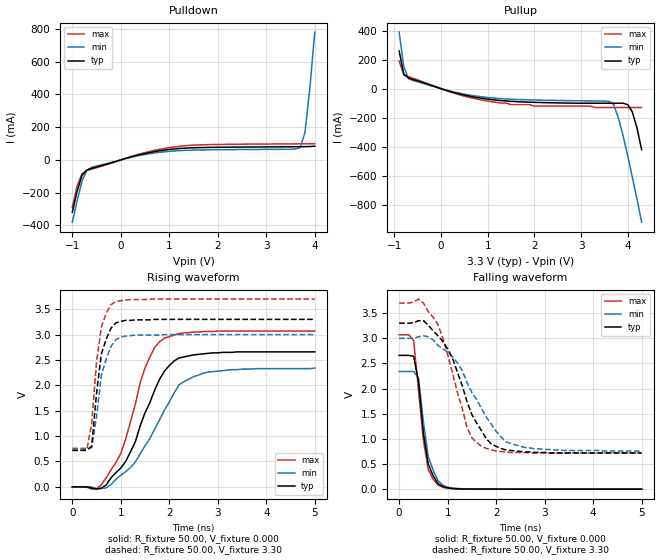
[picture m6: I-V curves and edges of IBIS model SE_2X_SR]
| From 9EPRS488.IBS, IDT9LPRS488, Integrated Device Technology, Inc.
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|   Model SE_2X_SR
[Model]   SE_2X_SR
Model_type   Output
Polarity   Inverting
Vmeas =   1.50V
Cref =   5.00pF
Rref =  0.000
Vref =   1.50V
C_comp   3.40pF   2.85pF   3.95pF
[Temperature Range]   27.00   70.00   0.000
[Voltage Range]   3.30V   3.00V   3.70V
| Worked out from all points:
|   slope of the pulldown table from 0 to 0.495 V, typ, clamps not added: 12.7 ohm
|   slope of the pullup table from 0 to 0.495 V, typ, clamps not added: 11.3 ohm
|   rising waveform, R_fixture 50.00, V_fixture 0.000: 20-80 % time 688ps typ, 834ps min, 578ps max; typ from 0 V to 2.66 V
|   rising waveform, R_fixture 50.00, V_fixture 3.30: 20-80 % time 215ps typ, 241ps min, 187ps max; typ from 0.72 V to 3.3 V
|   falling waveform, R_fixture 50.00, V_fixture 0.000: 20-80 % time 195ps typ, 229ps min, 211ps max; typ from 2.66 V to 0 V
|   falling waveform, R_fixture 50.00, V_fixture 3.30: 20-80 % time 646ps typ, 794ps min, 514ps max; typ from 3.3 V to 0.72 V
[Pulldown]
| voltage   I(typ)   I(min)   I(max)
|  -3.30   -4.16A   -4.01A   -4.26A
|  -3.10   -3.82A   -3.69A   -3.90A
|  -2.90   -3.48A   -3.37A   -3.55A
|  -2.70   -3.14A   -3.05A   -3.20A
|  -2.50   -2.80A   -2.72A   -2.85A
|  -2.30   -2.46A   -2.41A   -2.50A
|  -2.10   -2.12A   -2.09A   -2.15A
|  -1.90   -1.79A   -1.77A   -1.80A
|  -1.70   -1.45A   -1.45A   -1.45A
|  -1.50   -1.12A   -1.14A   -1.11A
-1V       -320mA     -380mA     -290mA
-900mV    -190mA     -250mA     -160mA
-800mV    -94.75mA   -130mA     -84.77mA
-700mV    -60.71mA   -64.75mA   -65.52mA
-600mV    -51.06mA   -45.2mA    -56.5mA
400mV     32.6mA     27.52mA    37.03mA
1.2V      69.5mA     56.57mA    82.87mA
3.5V      80.08mA    65.45mA    97.87mA
3.7V      80.56mA    75.15mA    98.32mA
3.8V      80.96mA    170mA      98.58mA
3.9V      81.72mA    440mA      98.88mA
4V        83.73mA    780mA      99.22mA
|   4.10   0.11A   1.16A   99.62mA
|   4.20   0.31A   1.55A   0.10A
|   4.30   0.66A   1.95A   0.10A
|   4.50   1.46A   2.77A   0.11A
|   4.70   2.32A   3.60A   0.58A
|   4.90   3.19A   4.43A   1.41A
|   5.10   4.07A   5.27A   2.30A
|   5.30   4.96A   6.12A   3.20A
|   5.50   5.85A   6.96A   4.12A
|   5.70   6.75A   7.81A   5.04A
|   5.90   7.65A   8.66A   5.97A
|   6.10   8.55A   9.52A   6.90A
|   6.60   10.81A   11.65A   9.23A
[Pullup]
| voltage   I(typ)   I(min)   I(max)
|  -3.30   10.68A   10.27A   10.94A
|  -3.10   9.79A   9.43A   10.01A
|  -2.90   8.89A   8.58A   9.09A
|  -2.70   7.99A   7.73A   8.16A
|  -2.50   7.10A   6.88A   7.23A
|  -2.30   6.20A   6.04A   6.31A
|  -2.10   5.31A   5.20A   5.38A
|  -1.90   4.43A   4.36A   4.47A
|  -1.70   3.54A   3.53A   3.55A
|  -1.50   2.67A   2.70A   2.64A
|  -1.00   0.59A   0.73A   0.50A
-900mV    260mA      390mA      190mA
-800mV    98.15mA    150mA      96.76mA
-700mV    74.35mA    69.94mA    82.79mA
-600mV    63.81mA    56.49mA    71.52mA
500mV     -44.25mA   -37.82mA   -51.47mA
1.5V      -86.95mA   -72.42mA   -110mA
3.5V      -100mA     -85.41mA   -130mA
3.7V      -100mA     -110mA     -130mA
3.9V      -100mA     -320mA     -130mA
4.1V      -160mA     -610mA     -130mA
4.2V      -270mA     -760mA     -130mA
4.3V      -420mA     -920mA     -130mA
|   4.50   -0.73A   -1.22A   -0.15A
|   4.70   -1.06A   -1.54A   -0.40A
|   4.90   -1.39A   -1.86A   -0.73A
|   5.10   -1.72A   -2.17A   -1.06A
|   5.30   -2.06A   -2.49A   -1.41A
|   5.50   -2.40A   -2.81A   -1.75A
|   5.70   -2.74A   -3.13A   -2.10A
|   5.90   -3.07A   -3.46A   -2.45A
|   6.10   -3.41A   -3.78A   -2.80A
|   6.60   -4.27A   -4.58A   -3.68A
[Ramp]
| variable   typ   min   max
dV/dt_r   1.60/0.68n   1.40/0.86n   1.84/0.58n
dV/dt_f   1.55/0.65n   1.34/0.79n   1.79/0.52n
[Rising Waveform]
R_fixture = 50.00
V_fixture = 0.000
V_fixture_min = 0.000
V_fixture_max = 0.000
| time   V(typ)   V(min)   V(max)
0s        0V         1.34uV     0V
500ps     -41.77mV   -34.07mV   -37.65mV
900ps     280mV      150mV      480mV
1.2ns     690mV      380mV      1.28V
1.5ns     1.46V      810mV      2.34V
1.7ns     1.91V      1.14V      2.75V
1.9ns     2.28V      1.51V      2.93V
2.2ns     2.54V      2.01V      3.02V
2.7ns     2.62V      2.24V      3.06V
5ns       2.66V      2.34V      3.07V
[Rising Waveform]
R_fixture = 50.00
V_fixture = 3.30
V_fixture_min = 3.00
V_fixture_max = 3.70
| time   V(typ)   V(min)   V(max)
0s        720mV      760mV      720mV
300ps     720mV      760mV      730mV
400ps     800mV      770mV      1.24V
500ps     1.84V      1.38V      2.46V
600ps     2.62V      2.2V       3.15V
700ps     2.91V      2.52V      3.42V
800ps     3.13V      2.77V      3.59V
900ps     3.23V      2.9V       3.65V
1.3ns     3.29V      2.99V      3.69V
5ns       3.3V       3V         3.7V
[Falling Waveform]
R_fixture = 50.00
V_fixture = 0.000
V_fixture_min = 0.000
V_fixture_max = 0.000
| time   V(typ)   V(min)   V(max)
0s        2.66V      2.34V      3.07V
200ps     2.66V      2.34V      3.07V
300ps     2.64V      2.34V      2.95V
400ps     2.13V      2.21V      1.96V
500ps     1.11V      1.34V      970mV
600ps     500mV      650mV      390mV
800ps     110mV      170mV      85.62mV
1ns       26.62mV    38.93mV    18.32mV
1.3ns     3.92mV     7.72mV     2.73mV
5ns       2.87uV     8.53uV     0V
[Falling Waveform]
R_fixture = 50.00
V_fixture = 3.30
V_fixture_min = 3.00
V_fixture_max = 3.70
| time   V(typ)   V(min)   V(max)
0s        3.3V       3V         3.7V
400ps     3.35V      3.03V      3.78V
800ps     3.05V      2.86V      3.27V
1.1ns     2.6V       2.63V      2.31V
1.4ns     1.74V      2.12V      1.23V
1.7ns     1.16V      1.6V       850mV
1.9ns     900mV      1.29V      780mV
2.2ns     780mV      940mV      740mV
2.5ns     750mV      850mV      730mV
5ns       720mV      760mV      720mV
